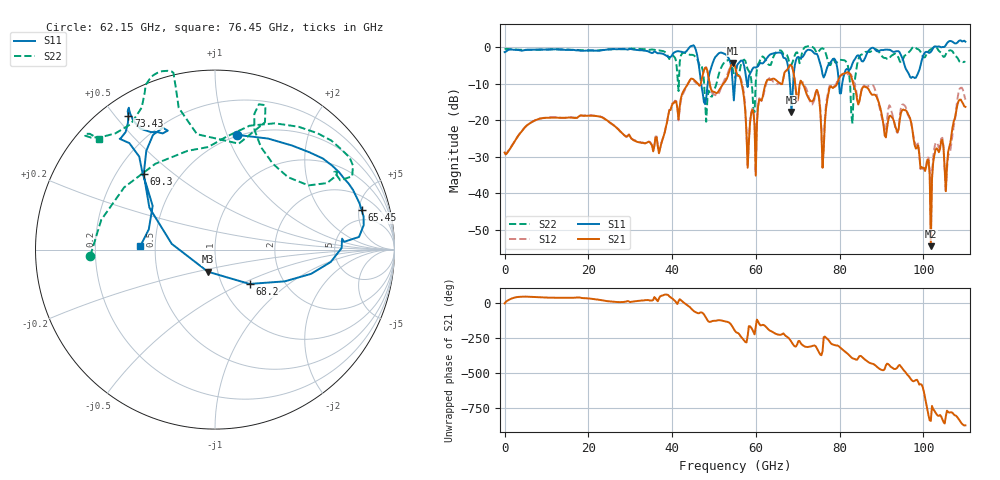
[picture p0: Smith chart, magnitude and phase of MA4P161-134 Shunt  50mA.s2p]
!Keysight Technologies,N5247B,US61255204,A.15.70.20
!Date: Friday, October 21, 2022 14:15:26
!Correction: S11(C  4-Port  )
!S31(C  4-Port  )
!S13(C  4-Port  )
!S33(C  4-Port  )
!S2P File: Measurements: S11, S31, S13, S33:
# Hz S  dB  R 50
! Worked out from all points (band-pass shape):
!   401 points, 10 MHz to 110 GHz, reference 50 ohm
!   highest |S21| = -4.28 dB at 54.46 GHz (marker M1); lowest = -54.5 dB at 101.8 GHz (marker M2)
!   |S21| within 3 dB of the highest: 53.46 GHz to 55.46 GHz (1.991 GHz wide, 3.66 % of centre); 66.76 GHz to 69.03 GHz (2.274 GHz wide, 3.35 % of centre)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
!   lowest |S11| = -17.8 dB at 68.48 GHz (marker M3), VSWR 1.30, Z = 44.9 - j11.2 ohm
!   |S11| at or under -10 dB: 46.94 GHz to 48.5 GHz (1.558 GHz wide, 3.26 % of centre); 68.11 GHz to 68.88 GHz (767.2 MHz wide, 1.12 % of centre); 79.83 GHz to 80.59 GHz (752.3 MHz wide, 0.938 % of centre)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
!   |S22| runs from -21.0 to 0.3 dB; largest |S21 - S12| = 0.16
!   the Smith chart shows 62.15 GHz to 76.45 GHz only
!   S11 on the Smith chart (normalised r, x): 62.15 GHz: 0.49, +1.09; 65.45 GHz: 3.45, +5.36; 68.2 GHz: 1.35, -0.56; 69.3 GHz: 0.31, +0.39; 73.43 GHz: 0.08, +0.54; 76.45 GHz: 0.41, +0.02
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1e7  -1.32 -179.9  -28.86 -3.5  -28.86 -3.1  -0.44 -180.0
1.843332e10  -0.93 130.7  -18.69 34.6  -18.71 34.4  -0.78 140.5
3.685665e10  -1.62 126.4  -29.07 32.0  -28.88 31.9  -0.86 133.9
4.565585e10  -0.69 52.3  -9.39 -67.4  -9.77 -65.9  -2.70 27.4
4.84056e10  -10.79 138.7  -6.43 -122.7  -6.33 -122.4  -14.31 128.3
5.445505e10  -9.90 98.0  -4.28 -173.4  -4.34 -173.3  -5.89 127.7
5.5005e10  -10.17 -177.3  -5.26 159.3  -5.47 158.9  -8.28 147.7
5.802972e10  -10.90 160.1  -33.03 123.4  -32.83 122.7  -6.08 167.5
6.215435e10  -3.73 79.0  -10.62 -164.4  -11.33 -159.1  -3.15 -177.2
6.545405e10  -1.45 15.1  -9.66 132.4  -9.71 154.2  -0.93 38.5
6.82038e10  -11.33 -44.8  -4.81 94.0  -4.97 91.0  -4.84 44.8
6.847878e10  -17.75 -107.8  -4.97 80.7  -5.17 78.3  -4.78 56.0
6.93037e10  -4.77 133.4  -9.48 48.6  -9.22 47.9  -2.08 73.8
7.342832e10  -1.03 122.9  -14.86 52.0  -15.70 50.1  0.12 111.2
7.645305e10  -7.62 177.2  -20.72 119.0  -19.72 130.7  -0.98 136.4
8.085265e10  -8.35 -75.6  -7.23 21.7  -7.66 22.0  -3.49 -144.1
8.305245e10  -4.42 -45.5  -9.27 -35.9  -8.72 -19.9  -20.95 16.7
8.607718e10  -2.85 6.5  -10.86 -46.5  -10.71 -45.4  -1.29 -14.6
9.185165e10  -0.68 71.7  -18.85 -85.2  -15.90 -82.2  -3.02 67.1
9.762612e10  -8.21 177.3  -25.10 159.5  -24.64 157.6  0.14 166.1
1.017508e11  -1.27 -88.1  -54.54 -123.8  -51.67 -113.4  -0.53 -124.4
1.1e11  1.53 8.3  -16.34 -155.5  -14.37 -160.8  -4.04 16.1
